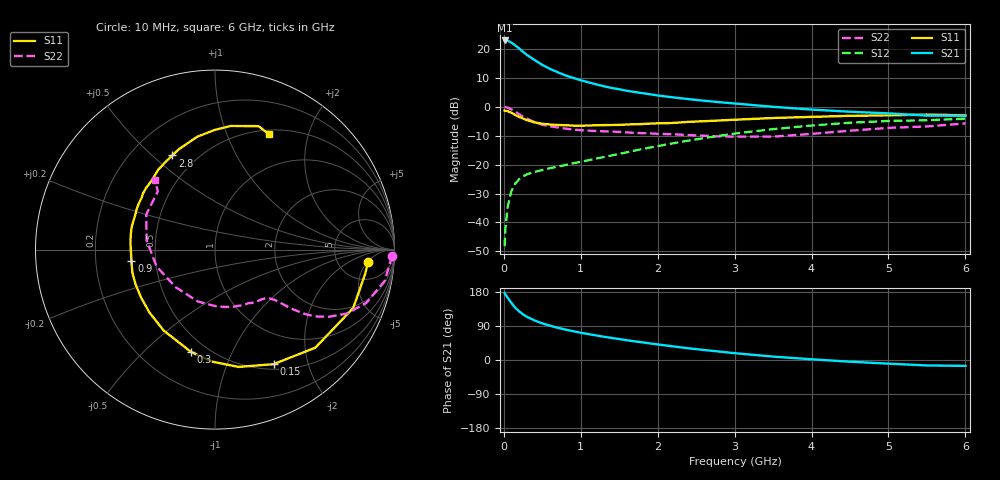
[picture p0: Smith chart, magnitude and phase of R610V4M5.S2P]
! SIEMENS Small Signal Semiconductors
! BFR193
! Si NPN RF Bipolar Junction Transistor in SOT23
! VCE = 10 V  IC = 4.5 mA
! Common Emitter S-Parameters:  May  1996
# GHz  S  MA  R  50
!  f  S11  S21  S12  S22
! GHz  MAG  ANG  MAG  ANG  MAG  ANG  MAG  ANG
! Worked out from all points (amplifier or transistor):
!   36 points, 10 MHz to 6 GHz, reference 50 ohm
!   highest |S21| = 22.9 dB at 10 MHz (marker M1)
!   |S21| within 3 dB of that: start of sweep to 210.1 MHz
!   unconditionally stable (mu >= 1): 957.9 MHz to 2.084 GHz
!   at 250 MHz: K = 0.39, MSG = 21.5 dB, |S12| = -24.1 dB
!   at 1.4 GHz: K = 1.07, MAG = 10.0 dB, |S12| = -16.9 dB
!   at 6 GHz: K = 0.96, MSG = 0.5 dB, |S12| = -4.2 dB
!   S11 on the Smith chart (normalised r, x): 10 MHz: 10, -5; 150 MHz: 0.56, -1.48; 300 MHz: 0.41, -0.71; 900 MHz: 0.36, -0.06; 2.8 GHz: 0.37, +0.58; 6 GHz: 0.55, +1.43
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0.01  0.8558 -4.6  13.89 176.9  0.0039 81.8  0.989 -2.0
0.02  0.8473 -9.3  13.85 173.4  0.0077 84.6  0.9788 -4.2
0.05  0.836 -22.9  13.79 164.2  0.0189 76.9  0.9618 -10.4
0.1  0.7819 -44.3  12.68 150.3  0.0353 67.8  0.894 -19.4
0.15  0.717 -62.9  11.36 137.5  0.0474 60.2  0.8159 -25.9
0.2  0.6667 -78.7  10.11 128.1  0.056 55.1  0.7358 -30.6
0.25  0.6234 -91.9  8.808 120.3  0.0627 51.1  0.6711 -33.7
0.3  0.5854 -103.2  7.821 114.0  0.0678 48.6  0.6205 -35.5
0.4  0.5341 -122.3  6.376 104.4  0.0748 46.7  0.539 -37.7
0.5  0.5066 -136.0  5.259 96.6  0.0805 46.2  0.4872 -38.8
0.6  0.491 -147.0  4.485 90.5  0.0867 46.8  0.4581 -39.3
0.7  0.483 -156.4  3.928 85.1  0.0921 48.2  0.4363 -40.1
0.9  0.4704 -172.0  3.14 76.0  0.105 51.5  0.4013 -42.2
1.1  0.4724 175.8  2.625 68.3  0.1187 54.5  0.3852 -45.3
1.3  0.4802 165.6  2.251 61.4  0.1351 56.6  0.3747 -48.9
1.6  0.4916 152.5  1.877 52.1  0.1629 58.6  0.3596 -55.8
2.2  0.5228 132.1  1.446 35.9  0.233 58.1  0.3334 -73.7
2.8  0.5762 114.4  1.194 22.3  0.314 52.7  0.3064 -98.6
3.5  0.636 99.1  0.993 9.0  0.409 42.5  0.3032 -136.4
4.5  0.6942 82.8  0.817 -4.5  0.5273 25.8  0.3838 172.5
5.5  0.7294 70.6  0.7 -14.4  0.5823 8.2  0.4551 134.4
6  0.7099 64.9  0.694 -15.5  0.62 3.3  0.5134 130.7
